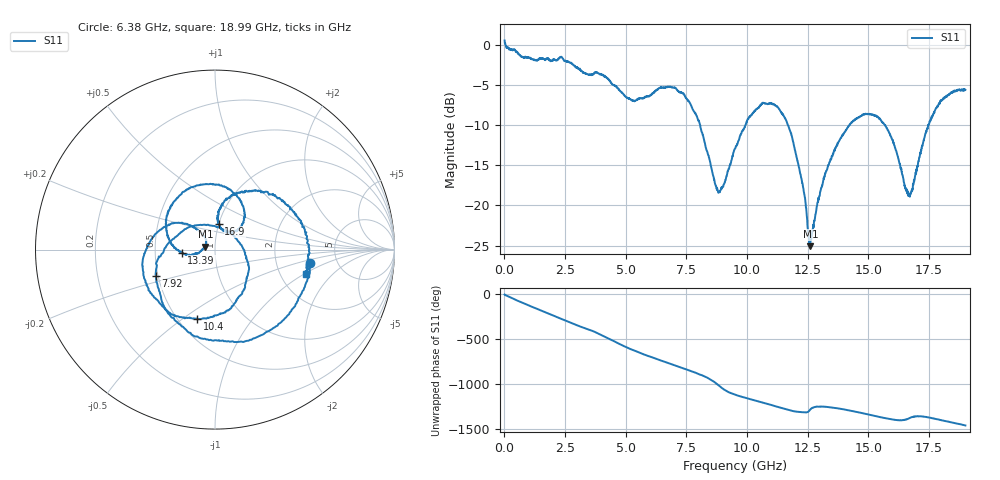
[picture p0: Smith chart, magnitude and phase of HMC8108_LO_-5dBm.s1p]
! Analog Devices, Inc.
! 1 Analog Way
! Wilmington, MA 01887
! http://www.analog.com
! Date:  2021-09-07 NN
! Board Name:  EV1HMC8108LC5 Revision A with HMC8108LC5 installed
! File Description:  S-Parameters for evaluation board without connectors or board loss de-embedded
! File Generation:  Calibrated Network Analyzer
! Chip Part Number:  HMC8108
! Chip Description:  X-Band, GaAs, MMIC, Low Noise Converter
! Chip Frequency:  9 to 10 GHz
! Chip Package:  LCC, 5 x 5 x 1.12 mm
! Chip State:
!  Temperature:  25C
!  LO Power:  -5dBm
! Note:
!  Analog Devices supplies this data as a sample of measured data at the evaluation board
!  ports for this product.  Your particular data for this product may vary.
!  Analog Devices reserves the right to change this data at anytime.
!  All lines below in this file are as is from the Network Analyzer.
!Keysight Technologies,N5245A,MY49151104,A.10.65.16
!Date: Wednesday, August 25, 2021 16:22:33
!Correction: S11(Full 2 Port(1,2))
!S1P File: Measurement: S11:
# Hz S  dB  R 50
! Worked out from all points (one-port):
!   1900 points, 10 MHz to 19 GHz, reference 50 ohm
!   lowest |S11| = -25.1 dB at 12.61 GHz (marker M1), VSWR 1.12, Z = 44.9 + j1.52 ohm
!   |S11| at or under -10 dB: 8.066 GHz to 9.936 GHz (1.87 GHz wide, 20.8 % of centre); 11.68 GHz to 14.21 GHz (2.528 GHz wide, 19.5 % of centre); 15.68 GHz to 17.47 GHz (1.791 GHz wide, 10.8 % of centre)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
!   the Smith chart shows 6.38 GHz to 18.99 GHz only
!   S11 on the Smith chart (normalised r, x): 6.38 GHz: 3.17, -0.66; 7.92 GHz: 0.49, -0.17; 10.4 GHz: 0.62, -0.57; 13.39 GHz: 0.69, -0.03; 16.9 GHz: 1.00, +0.29; 18.99 GHz: 2.78, -1.05
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1e7  0.53 -2.0
6.1e8  -1.22 -78.6
9.7e8  -1.57 -118.6
1.43e9  -1.82 -169.8
1.83e9  -1.78 145.3
2.39e9  -1.65 82.8
3.06e9  -3.00 10.1
3.86e9  -3.54 -74.2
4.34e9  -4.51 -137.4
4.76e9  -5.77 166.3
5.51e9  -6.79 78.9
6.38e9  -5.40 -8.0
7.14e9  -5.70 -81.0
7.92e9  -8.85 -155.6
8.82e9  -18.43 71.0
9.51e9  -12.90 -35.3
1.04e10  -7.97 -104.3
1.118e10  -7.57 -163.8
1.188e10  -11.83 144.5
1.261e10  -25.07 162.4
1.339e10  -14.63 -174.2
1.426e10  -9.85 147.5
1.555e10  -9.57 72.0
1.663e10  -18.43 58.1
1.69e10  -16.78 81.9
1.791e10  -7.27 48.1
1.899e10  -5.57 -15.0
1.9e10  -5.61 -16.8
